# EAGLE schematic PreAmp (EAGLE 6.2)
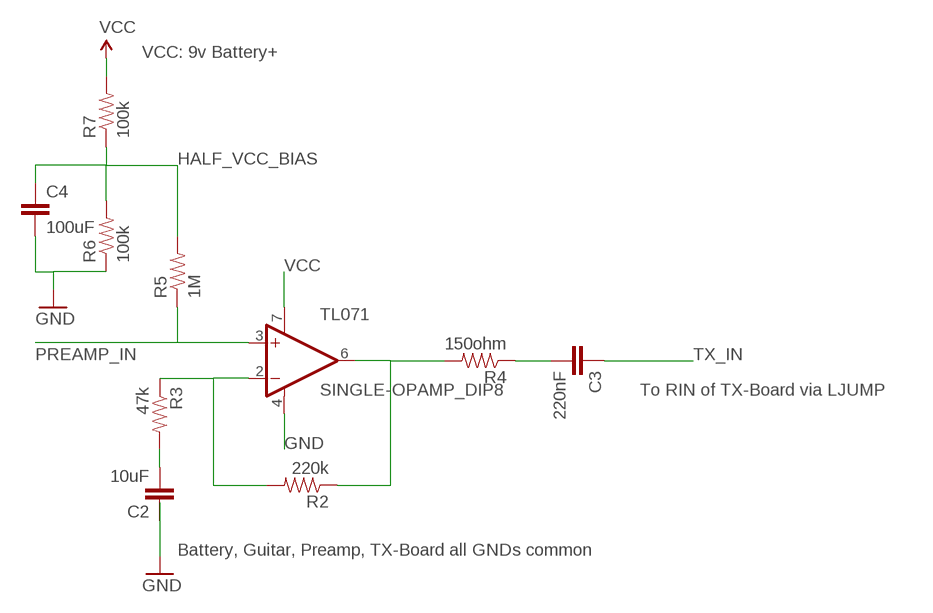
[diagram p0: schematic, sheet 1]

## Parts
C2  10uF  CAPPTH  [CAP-PTH-SMALL]
C3  220nF  CAPPTH  [CAP-PTH-SMALL]
C4  100uF  CAPPTH  [CAP-PTH-SMALL]
R2  220k  RESISTORAXIAL-0.3  [AXIAL-0.3]
R3  47k  RESISTORAXIAL-0.3  [AXIAL-0.3]
R4  150ohm  RESISTORAXIAL-0.3  [AXIAL-0.3]
R5  1M  RESISTORAXIAL-0.3  [AXIAL-0.3]
R6  100k  RESISTORAXIAL-0.3  [AXIAL-0.3]
R7  100k  RESISTORAXIAL-0.3  [AXIAL-0.3]
TL071  SINGLE-OPAMP_DIP8  [DIP-8]

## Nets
GND: C4.2 R6.P$1 TL071.4(V-)
HALF_VCC_BIAS: C4.1 R5.P$2 R6.P$2 R7.P$1
N$1: R2.P$2 R3.P$1 TL071.2(-IN)
N$2: R2.P$1 R4.P$2 TL071.6(OUT)
N$3: C2.2 R3.P$2
N$4: C3.2 R4.P$1
PREAMP_IN: R5.P$1 TL071.3(+IN)
TX_IN: C3.1
VCC: R7.P$2 TL071.7(V+)
Unconnected: C2.1

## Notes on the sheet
- VCC: 9v Battery+
- To RIN of TX-Board via LJUMP
- Battery, Guitar, Preamp, TX-Board all GNDs common

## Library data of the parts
C2-C4 = SparkFun-Passives:CAP: Capacitor
R2-R7 = SparkFun-Passives:RESISTOR: Resistor
TL071 = opamps:SINGLE-OPAMP: Generic single-channel op-amp

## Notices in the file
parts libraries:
SparkFun-Passives: Licensing: CC v3.0 Share-Alike You are welcome to use this library for commercial purposes.
